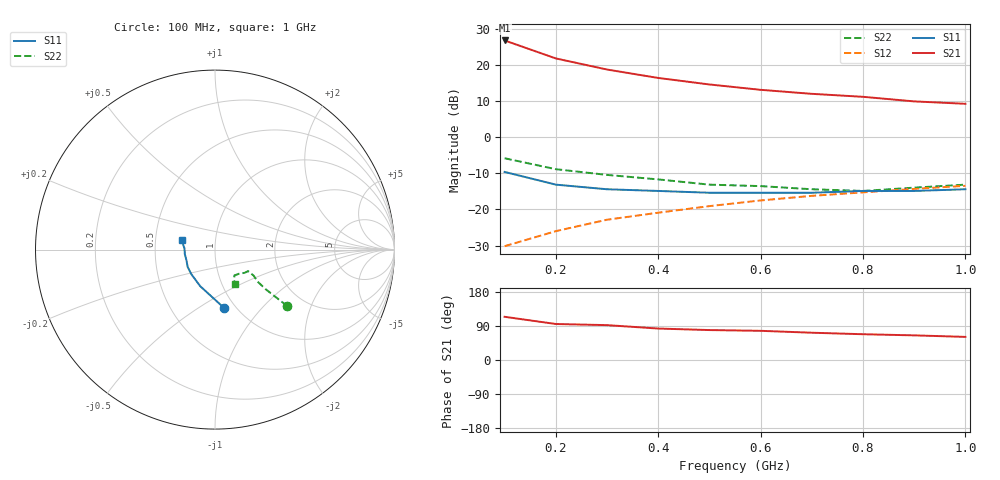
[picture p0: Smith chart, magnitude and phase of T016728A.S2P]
!AT-01672
!S-PARAMETERS at Vce=8V  Ic=35mA.  LAST UPDATED 07-21-92
!OBSOLETED Feb 1994 - nearest replacement: AT-42070
# ghz s ma r 50
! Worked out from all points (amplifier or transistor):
!   10 points, 100 MHz to 1 GHz, reference 50 ohm
!   highest |S21| = 26.7 dB at 100 MHz (marker M1)
!   |S21| within 3 dB of that: start of sweep to 160.3 MHz
!   unconditionally stable (mu >= 1): 369.2 MHz to end of sweep
!   at 200 MHz: K = 0.92, MSG = 23.9 dB, |S12| = -26.0 dB
!   at 600 MHz: K = 1.04, MAG = 14.1 dB, |S12| = -17.5 dB
!   at 1 GHz: K = 1.02, MAG = 10.6 dB, |S12| = -13.5 dB
0.1  0.33 -81.0  21.73 114.0  0.031 72.0  0.51 -38.0
0.2  0.22 -112.0  12.26 95.0  0.05 75.0  0.36 -38.0
0.3  0.19 -134.0  8.61 92.0  0.072 74.0  0.3 -37.0
0.4  0.18 -148.0  6.58 83.0  0.09 72.0  0.26 -34.0
0.5  0.17 -159.0  5.35 79.0  0.111 70.0  0.22 -33.0
0.6  0.17 -171.0  4.51 77.0  0.133 71.0  0.21 -38.0
0.7  0.17 178.0  3.97 72.0  0.154 68.0  0.19 -45.0
0.8  0.18 171.0  3.61 68.0  0.172 66.0  0.18 -53.0
0.9  0.18 169.0  3.12 65.0  0.192 66.0  0.2 -58.0
1  0.19 164.0  2.89 61.0  0.212 63.0  0.22 -60.0
